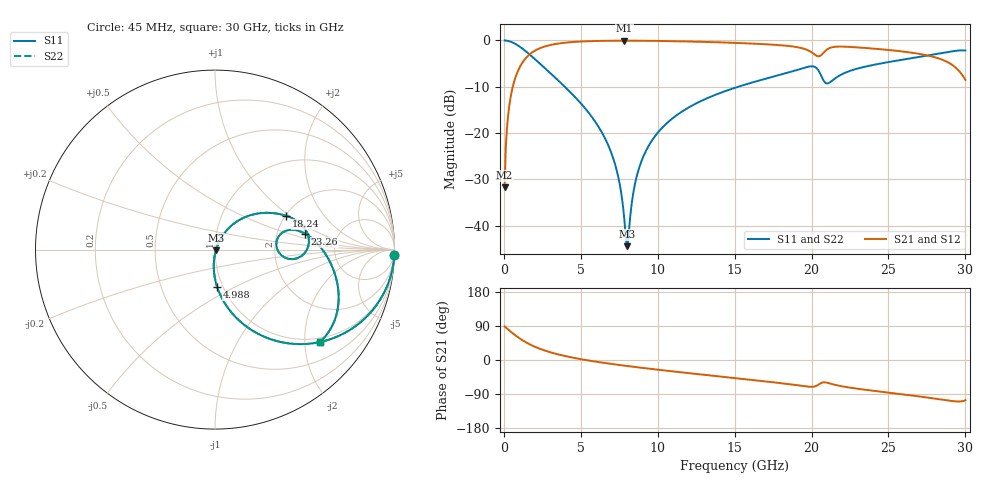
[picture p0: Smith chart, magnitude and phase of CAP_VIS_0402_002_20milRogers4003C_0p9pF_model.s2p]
! S-parameter model data by Modelithics Inc.  support@modelithics.com  813-866-6335  Tampa FL USA
! S-Parameter data specifications:
! Substrate: 20-mil Rogers 4003C, substrate thickness, H=0.508mm, Dielectric constant, Er=3.75
! PCB Mounting Pad Footprint: Pad width, PadW=0.50mm , Pad length, PadL=0.50mm , Pad gap, PadG (edge-to-edge)=0.40mm , Reference planes=1.4mm apart
! Created Wed Nov 18 12:38:17 2015
# hz S ma R 50
! 2 Port Network Data from SP1.SP block
! freq  magS11  angS11  magS21  angS21  magS12  angS12  magS22  angS22
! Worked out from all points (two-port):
!   401 points, 45 MHz to 30 GHz, reference 50 ohm
!   highest |S21| = -0.05 dB at 7.833 GHz (marker M1); lowest = -31.7 dB at 45 MHz (marker M2)
!   |S21| within 3 dB of the highest: 1.657 GHz to 20.21 GHz (18.55 GHz wide, 170 % of centre); 20.66 GHz to 27.26 GHz (6.592 GHz wide, 27.5 % of centre)
!   lowest |S11| = -44.4 dB at 7.983 GHz (marker M3), VSWR 1.01, Z = 50.5 - j0.306 ohm
!   |S11| at or under -10 dB: 3.958 GHz to 15.23 GHz (11.27 GHz wide, 117 % of centre)
!   |S22| runs from -44.4 to 0.0 dB; largest |S21 - S12| = 0
!   S11 on the Smith chart (normalised r, x): 45 MHz: 1, -73; 4.988 GHz: 0.94, -0.41; 18.24 GHz: 2.02, +0.94; 23.26 GHz: 2.90, +0.69; 30 GHz: 0.90, -2.36
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4.5e7  0.9997 -1.6  0.02586 88.4  0.02586 88.4  0.9997 -1.6
2.696625e8  0.9881 -9.4  0.1533 80.6  0.1533 80.6  0.9881 -9.4
4.194375e8  0.9719 -14.4  0.2349 75.6  0.2349 75.6  0.9719 -14.4
1.168312e9  0.8241 -36.7  0.5651 53.2  0.5651 53.2  0.8241 -36.7
2.74095e9  0.489 -65.8  0.8693 23.8  0.8693 23.8  0.489 -65.8
4.987575e9  0.2104 -86.5  0.9731 2.3  0.9731 2.3  0.2104 -86.5
5.062462e9  0.2036 -87.0  0.9745 1.7  0.9745 1.7  0.2036 -87.0
7.009538e9  0.05931 -95.3  0.9926 -10.5  0.9926 -10.5  0.05931 -95.3
7.53375e9  0.02778 -91.7  0.9938 -13.4  0.9938 -13.4  0.02778 -91.7
7.8333e9  0.01147 -74.9  0.994 -14.9  0.994 -14.9  0.01147 -74.9
7.983075e9  0.006005 -30.3  0.9939 -15.7  0.9939 -15.7  0.006005 -30.3
8.806838e9  0.0429 61.9  0.9927 -19.9  0.9927 -19.9  0.0429 61.9
1.007992e10  0.1045 60.4  0.9876 -25.9  0.9876 -25.9  0.1045 60.4
1.50225e10  0.3082 40.5  0.9416 -47.8  0.9416 -47.8  0.3082 40.5
1.824266e10  0.4387 25.4  0.8803 -62.3  0.8803 -62.3  0.4387 25.4
2.003996e10  0.5259 6.0  0.7377 -70.8  0.7377 -70.8  0.5259 6.0
2.056418e10  0.4376 -7.0  0.6822 -62.1  0.6822 -62.1  0.4376 -7.0
2.10135e10  0.3429 4.1  0.8005 -59.9  0.8005 -59.9  0.3429 4.1
2.326012e10  0.5105 9.9  0.8349 -77.3  0.8349 -77.3  0.5105 9.9
2.505742e10  0.5862 1.5  0.7874 -86.3  0.7874 -86.3  0.5862 1.5
2.842736e10  0.7282 -19.1  0.6252 -104.3  0.6252 -104.3  0.7282 -19.1
3e10  0.7789 -41.3  0.3754 -106.0  0.3754 -106.0  0.7789 -41.3
